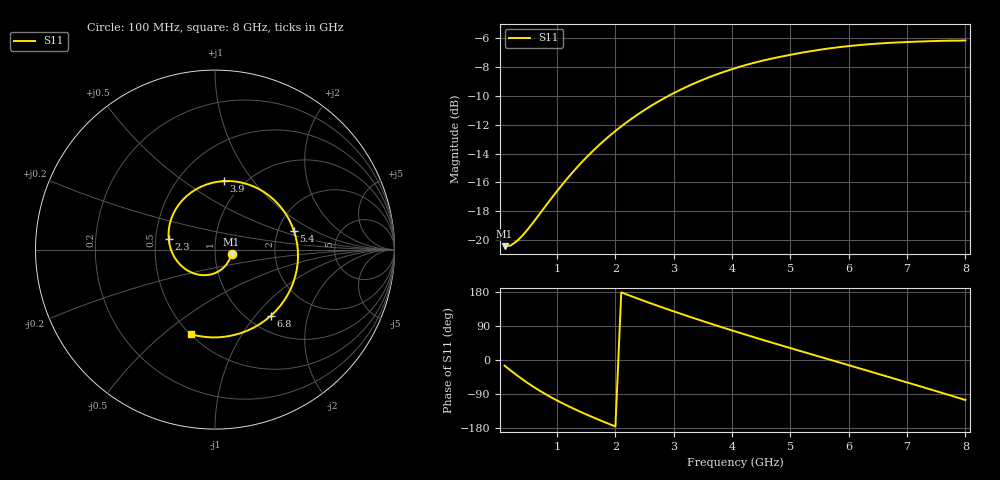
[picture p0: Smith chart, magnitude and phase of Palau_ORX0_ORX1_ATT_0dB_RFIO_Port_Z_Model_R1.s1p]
! Created Fri Oct  9 14:27:57 2020
! Palau ORX0/ORX1 RFIO Port Impedance Model.
! Attenuation  : 0 dB.
! Revision		: R1.
! Impedance Mode 	: Balanced Differential-Mode.
! Impedance Format 	: Series Equivalent Differential Impedance (SEDZ).
# hz S ma R 100
! 1 Port Network Data from SP1.SP block
! freq  magS11  angS11
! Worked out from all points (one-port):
!   80 points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, 100 MHz to 8 GHz, reference 100 ohm
!   lowest |S11| = -20.4 dB at 100 MHz (marker M1), VSWR 1.21, Z = 120 - j6.02 ohm
!   |S11| at or under -10 dB: start of sweep to 2.917 GHz
!   S11 on the Smith chart (normalised r, x): 100 MHz: 1.20, -0.06; 2.3 GHz: 0.59, +0.08; 3.9 GHz: 0.81, +0.73; 5.4 GHz: 2.45, +0.64; 6.8 GHz: 1.25, -1.21; 8 GHz: 0.51, -0.63
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1e8  0.09551 -15.1
2e8  0.09596 -27.2
4e8  0.1036 -50.4
8e8  0.1312 -90.0
1.1e9  0.1569 -114.7
1.3e9  0.175 -129.6
1.6e9  0.2025 -150.2
1.9e9  0.2298 -169.3
2.1e9  0.2477 178.5
2.3e9  0.2652 166.8
2.7e9  0.2989 144.4
3.1e9  0.3303 123.0
3.5e9  0.3589 102.6
3.9e9  0.3845 82.9
4.1e9  0.3961 73.2
4.3e9  0.4068 63.7
4.6e9  0.4211 49.7
4.8e9  0.4296 40.5
5.1e9  0.4415 26.9
5.4e9  0.4522 13.3
5.8e9  0.4641 -4.7
6.1e9  0.4712 -18.3
6.4e9  0.4769 -31.8
6.8e9  0.4825 -50.1
7.1e9  0.4853 -63.7
7.4e9  0.4877 -77.6
7.6e9  0.489 -86.8
8e9  0.4905 -105.5
